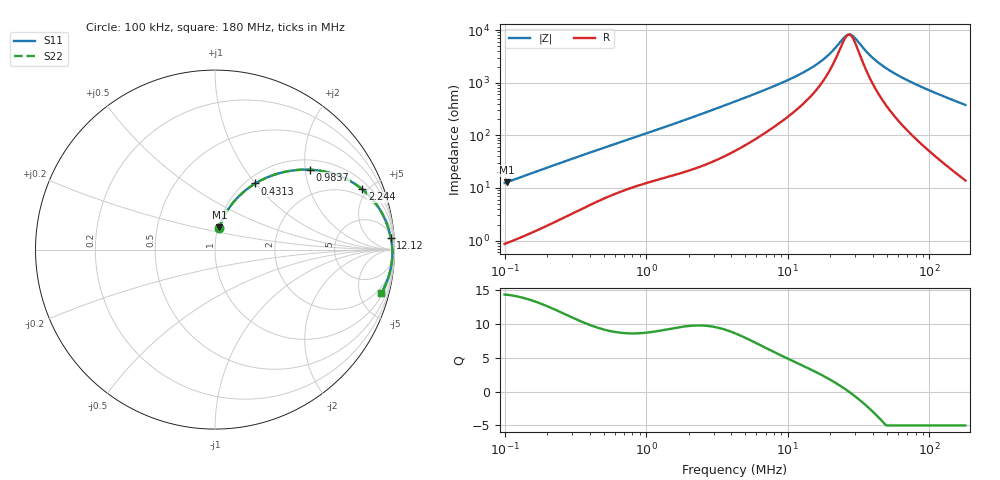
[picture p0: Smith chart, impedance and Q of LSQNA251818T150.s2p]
! LSQNA251818T150  S-PARAMETER MODEL  ( General Type )
! Model Generated by TAIYO YUDEN Corporation (http://www.ty-top.com)
! Version 2.0
! TAIYO YUDEN Control No. 100810NF25SB-FKC
! Copyright(c) 2007 TAIYO YUDEN CO.,LTD. All Rights Reserved.
! Product Description (link to TY-COMPAS)
! https://ds.yuden.co.jp/TYCOMPAS/or/detail?pn=LSQNA251818T150K&u=M
! Products Name : Inductors
! Characteristics :
!  Inductance : 15 uH , SRF(min) : 23 MHz , DC Resistance(max) : 0.416 Ohm
!  Rated Current : Saturation :180 mA , Temp Rise : 650 mA (40 degC)
!  Case Size : 2.5 x 1.8 / 0.098 x 0.071 [mm/inch] , Thickness : 1.8 / 0.071 [mm/inch]
!  (Conditions: Temperature = 25 degC , DC Bias Current/Voltage = 0A / 0V)
! External Node Assignments :
!  1  o---GGG---o  2
! GND o---------o GND
! Frequency Range : 0.1MHz  -  180.004543MHz  [ 402 STEP ]
# MHz S RI R 50
! Freq[MHz].  S11 Real  S11 Imag  S21 Real  S21 Imag  S12 Real  S12 Imag  S22 Real  S22 Imag
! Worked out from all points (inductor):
!   401 points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, 100 kHz to 180 MHz, reference 50 ohm
!   read as one part in series: L = 19.6 uH near 103.8 kHz
!   highest Q = 14.3 at 103.8 kHz (marker M1), where L = 19.7 uH
!   self-resonance near 27.03 MHz
!   S11 on the Smith chart (normalised r, x): 100 kHz: 1.02, +0.25; 431.3 kHz: 1.10, +1.00; 983.7 kHz: 1.24, +2.12; 2.244 MHz: 1.47, +4.62; 12.12 MHz: 8, +28; 180 MHz: 1.28, -7.53
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0.1  0.0232 0.1198  0.9768 -0.1198  0.9768 -0.1198  0.0232 0.1198
0.103819  0.0246 0.124  0.9754 -0.124  0.9754 -0.124  0.0246 0.124
0.203822  0.0734 0.224  0.9266 -0.224  0.9266 -0.224  0.0734 0.224
0.350962  0.1692 0.3297  0.8308 -0.3297  0.8308 -0.3297  0.1692 0.3297
0.431301  0.2245 0.3685  0.7755 -0.3685  0.7755 -0.3685  0.2245 0.3685
0.663681  0.3713 0.4291  0.6287 -0.4291  0.6287 -0.4291  0.3713 0.4291
0.983697  0.5288 0.445  0.4712 -0.445  0.4712 -0.445  0.5288 0.445
1.231743  0.6199 0.433  0.3801 -0.433  0.3801 -0.433  0.6199 0.433
2.243586  0.8201 0.3364  0.1799 -0.3364  0.1799 -0.3364  0.8201 0.3364
4.322947  0.931 0.2018  0.069 -0.2018  0.069 -0.2018  0.931 0.2018
7.874131  0.968 0.111  0.032 -0.111  0.032 -0.111  0.968 0.111
12.11662  0.9793 0.0653  0.0207 -0.0653  0.0207 -0.0653  0.9793 0.0653
14.89024  0.9826 0.0471  0.0174 -0.0471  0.0174 -0.0471  0.9826 0.0471
18.64491  0.9854 0.0288  0.0146 -0.0288  0.0146 -0.0288  0.9854 0.0288
25.16353  0.9877 0.00553  0.0123 -0.00553  0.0123 -0.00553  0.9877 0.00553
27.12217  0.988 -0.000256  0.012 0.000256  0.012 0.000256  0.988 -0.000256
29.78622  0.9883 -0.00756  0.0117 0.00756  0.0117 0.00756  0.9883 -0.00756
35.25813  0.9885 -0.021  0.0115 0.021  0.0115 0.021  0.9885 -0.021
40.20007  0.9882 -0.032  0.0118 0.032  0.0118 0.032  0.9882 -0.032
52.25907  0.9866 -0.0559  0.0134 0.0559  0.0134 0.0559  0.9866 -0.0559
86.6749  0.977 -0.1138  0.023 0.1138  0.023 0.1138  0.977 -0.1138
180.0045  0.9265 -0.2432  0.0735 0.2432  0.0735 0.2432  0.9265 -0.2432
